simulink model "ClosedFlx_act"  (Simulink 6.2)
settings: Solver=ode45  StartTime=0.0  StopTime=50  RelTol=1e-3
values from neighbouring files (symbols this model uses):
  Kp = om^2*Iy/(l*T)    (= 0.554556771732)    [run.m]    (also in run3.m = 0.554540604935)
  Kr = 2*0.85*om*Iy/(l*T)    (= 1.03530256089)    [run.m]    (also in run3.m = 1.03527237908)
  wd = 7    [run.m]    (also in run3.m)
  wd2 = 16    [run.m]    (also in run3.m)
  wf = 9    [run.m]    (also in run3.m)
  wn = 7.4    [run.m]    (also in run3.m)
  wn2 = 16.8    [run.m]    (also in run3.m)
  zd = 0.2    [run.m]    (also in run3.m)
  zd2 = 0.2    [run.m]    (also in run3.m)
  zn = 0.02    [run.m]    (also in run3.m)
  zn2 = 0.015    [run.m]    (also in run3.m)
undefined symbols (not defined in the file or in its folder): Ava, Bva, Cva, Dva

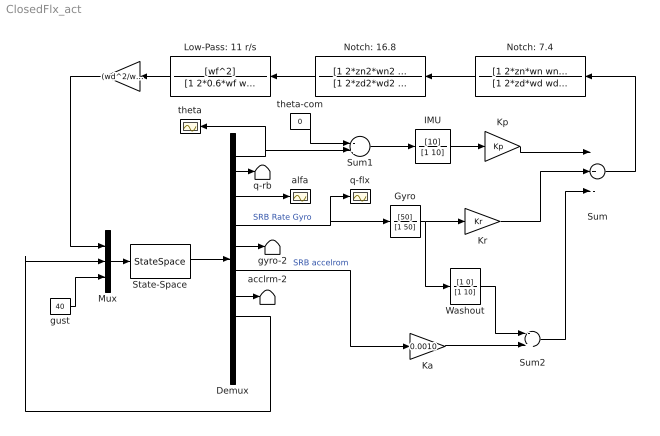
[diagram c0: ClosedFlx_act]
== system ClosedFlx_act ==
  " " : Gain  Orientation=left  Gain=(wd^2/wn^2)*(wd2^2/wn2^2)
  Demux : Demux  Outputs=10
  Gyro : TransferFcn  Numerator=[50]  Denominator=[1 50]
  IMU : TransferFcn  Numerator=[10]  Denominator=[1 10]
  Ka : Gain  Gain=0.0010
  Kp : Gain  Gain=Kp
  Kr : Gain  Gain=Kr
  Low-Pass: 11 r/s : TransferFcn  Orientation=left  Numerator=[wf^2]  Denominator=[1 2*0.6*wf wf^2]
  Mux : Mux  Inputs=3
  Notch: 16.8 : TransferFcn  Orientation=left  Numerator=[1 2*zn2*wn2 wn2^2]  Denominator=[1 2*zd2*wd2 wd2^2]
  Notch: 7.4 : TransferFcn  Orientation=left  Numerator=[1 2*zn*wn wn^2]  Denominator=[1 2*zd*wd wd^2]
  State-Space : StateSpace  A=Ava  B=Bva  C=Cva  D=Dva
  Sum : Sum  Inputs=++-
  Sum1 : Sum  Inputs=-+|
  Sum2 : Sum  Inputs=-+
  Washout : TransferFcn  Numerator=[1 0]  Denominator=[1 10]
  acclrm-2 : Terminator
  alfa : Scope
  gust : Constant  Value=40
  gyro-2 : Terminator
  q-flx : Scope
  q-rb : Terminator
  theta : Scope
  theta-com : Constant  Value=0
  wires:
  Mux/1 -> State-Space/1
  Demux/4 -> Gyro/1, q-flx/1  "SRB Rate Gyro"
  Demux/6 -> Ka/1  "SRB accelrom"
  Kp/1 -> Sum/1
  Kr/1 -> Sum/2
  Demux/7 -> acclrm-2/1
  Ka/1 -> Sum2/2
  Sum2/1 -> Sum/3
  State-Space/1 -> Demux/1
  Demux/2 -> q-rb/1
  Demux/3 -> alfa/1
  Demux/5 -> gyro-2/1
  IMU/1 -> Kp/1
  Gyro/1 -> Washout/1, Kr/1
  Demux/8 -> Mux/2
  gust/1 -> Mux/3
  Low-Pass: 11 r/s/1 -> " "/1
  " "/1 -> Mux/1
  Sum/1 -> Notch: 7.4/1
  Notch: 7.4/1 -> Notch: 16.8/1
  Notch: 16.8/1 -> Low-Pass: 11 r/s/1
  Demux/1 -> Sum1/2, theta/1
  Sum1/1 -> IMU/1
  theta-com/1 -> Sum1/1
  Washout/1 -> Sum2/1
